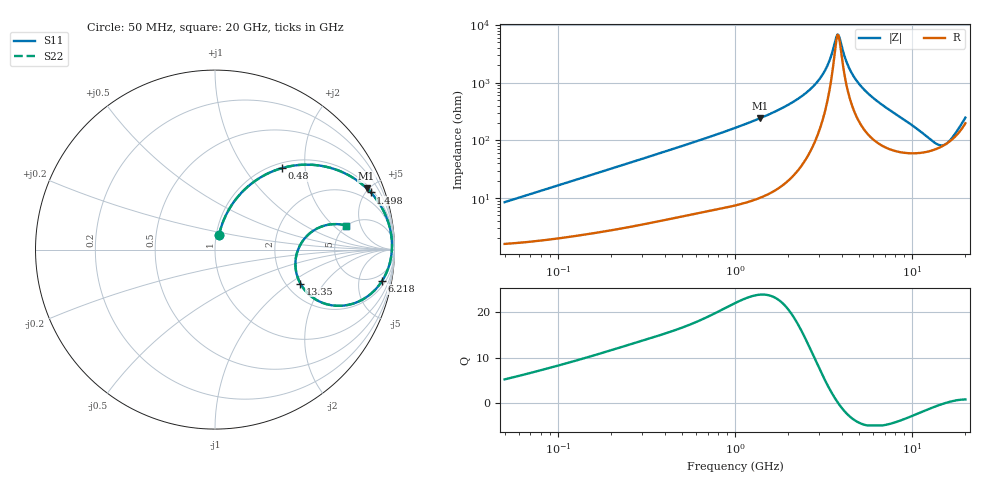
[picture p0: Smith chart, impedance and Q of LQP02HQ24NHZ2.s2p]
!Murata Part Number: LQP02HQ24NHZ2
!These Parameters are Measured in Series Mode Connection
!  o--[Z]--o
!Port1  Port2
!  o-------o
!Freq. Start=50[MHz] Stop=20[GHz], 401[Steps]
# Hz S RI R 50
!Freq.(Hz) S11(Real) S11(Imag) S21(Real) S21(Imag) S12(Real) S12(Imag) S22(Real) S22(Imag)
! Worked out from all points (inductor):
!   401 points, 50 MHz to 20 GHz, reference 50 ohm
!   read as one part in series: L = 26.4 nH near 51.52 MHz
!   highest Q = 23.9 at 1.39 GHz (marker M1), where L = 27.8 nH
!   self-resonance near 3.793 GHz
!   S11 on the Smith chart (normalised r, x): 50 MHz: 1.03, +0.17; 480 MHz: 1.09, +1.52; 1.498 GHz: 1.22, +5.35; 6.218 GHz: 3, -10; 13.35 GHz: 2.38, -1.22; 20 GHz: 4.96, +2.97
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5e7  0.0223 0.0801  0.9777 -0.0801  0.9777 -0.0801  0.0223 0.0801
1.364002e8  0.0663 0.2026  0.9337 -0.2026  0.9337 -0.2026  0.0663 0.2026
3.721004e8  0.2729 0.4131  0.7271 -0.4131  0.7271 -0.4131  0.2729 0.4131
4.800071e8  0.3745 0.4544  0.6255 -0.4544  0.6255 -0.4544  0.3745 0.4544
1e9  0.7198 0.427  0.2802 -0.427  0.2802 -0.427  0.7198 0.427
1.390315e9  0.8448 0.3419  0.1552 -0.3419  0.1552 -0.3419  0.8448 0.3419
1.498439e9  0.8675 0.3187  0.1325 -0.3187  0.1325 -0.3187  0.8675 0.3187
2.114743e9  0.9447 0.2042  0.0553 -0.2042  0.0553 -0.2042  0.9447 0.2042
2.728004e9  0.9753 0.1164  0.0247 -0.1164  0.0247 -0.1164  0.9753 0.1164
3.265178e9  0.985 0.0543  0.015 -0.0543  0.015 -0.0543  0.985 0.0543
3.792786e9  0.9857 0.00219  0.0143 -0.00219  0.0143 -0.00219  0.9857 0.00219
3.908127e9  0.9851 -0.00828  0.0149 0.00828  0.0149 0.00828  0.9851 -0.00828
4.275624e9  0.9813 -0.0399  0.0187 0.0399  0.0187 0.0399  0.9813 -0.0399
4.677679e9  0.9748 -0.0718  0.0252 0.0718  0.0252 0.0718  0.9748 -0.0718
5.273168e9  0.961 -0.1149  0.039 0.1149  0.039 0.1149  0.961 -0.1149
6.217679e9  0.9306 -0.175  0.0694 0.175  0.0694 0.175  0.9306 -0.175
7.442007e9  0.8762 -0.2394  0.1238 0.2394  0.1238 0.2394  0.8762 -0.2394
1.066139e10  0.6599 -0.3116  0.3401 0.3116  0.3401 0.3116  0.6599 -0.3116
1.334722e10  0.4761 -0.1897  0.5239 0.1897  0.5239 0.1897  0.4761 -0.1897
1.573793e10  0.4703 0.0169  0.5297 -0.0169  0.5297 -0.0169  0.4703 0.0169
1.774144e10  0.5854 0.1253  0.4146 -0.1253  0.4146 -0.1253  0.5854 0.1253
2e10  0.7309 0.134  0.2691 -0.134  0.2691 -0.134  0.7309 0.134
